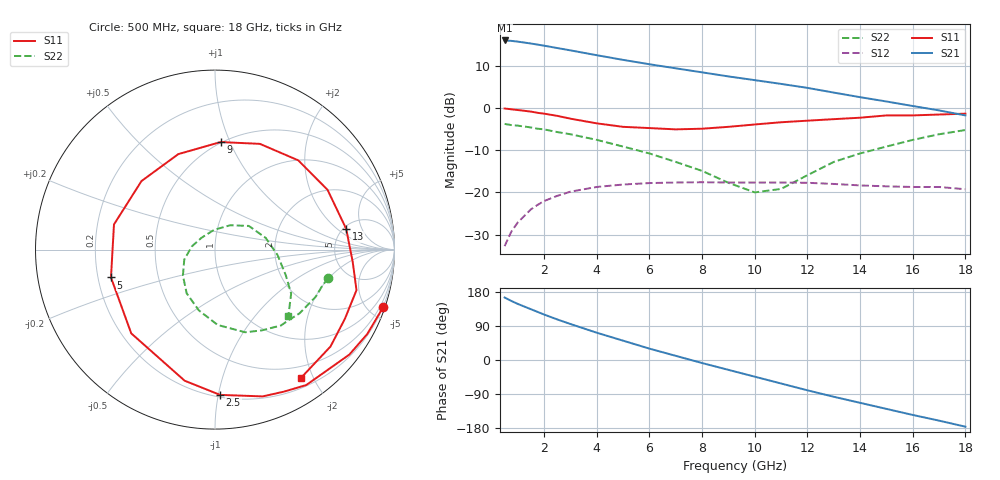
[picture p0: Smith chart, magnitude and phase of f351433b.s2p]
!ATF-35143
!S-PARAMETERS at Vds=3V  Id=10mA.  LAST UPDATED 06-3-99
# ghz s ma r 50
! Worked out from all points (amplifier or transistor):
!   23 points, 500 MHz to 18 GHz, reference 50 ohm
!   highest |S21| = 16.1 dB at 500 MHz (marker M1)
!   |S21| within 3 dB of that: start of sweep to 3.563 GHz
!   unconditionally stable (mu >= 1): 7.966 GHz to end of sweep
!   at 1.5 GHz: K = 0.23, MSG = 19.7 dB, |S12| = -24.0 dB
!   at 7 GHz: K = 0.91, MSG = 13.6 dB, |S12| = -17.7 dB
!   at 18 GHz: K = 1.40, MAG = 5.0 dB, |S12| = -19.3 dB
!   lowest NFmin = 0.12 dB at 500 MHz
!   S11 on the Smith chart (normalised r, x): 500 MHz: 0.18, -5.97; 2.5 GHz: 0.21, -1.01; 5 GHz: 0.25, -0.12; 9 GHz: 0.49, +0.92; 13 GHz: 5.27, +2.70; 18 GHz: 0.33, -1.83
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0.5  0.99 -19.0  6.36 165.0  0.023 77.0  0.65 -14.0
0.75  0.97 -29.0  6.29 156.0  0.034 70.0  0.63 -19.0
1  0.95 -38.0  6.16 148.0  0.044 65.0  0.62 -25.0
1.5  0.91 -56.0  5.85 134.0  0.063 54.0  0.59 -37.0
1.75  0.88 -64.0  5.68 127.0  0.071 49.0  0.57 -43.0
2  0.86 -72.0  5.51 120.0  0.079 44.0  0.56 -49.0
2.5  0.81 -88.0  5.17 107.0  0.091 35.0  0.52 -60.0
3  0.75 -103.0  4.85 95.0  0.102 26.0  0.49 -70.0
4  0.66 -135.0  4.25 72.0  0.116 10.0  0.42 -88.0
5  0.6 -165.0  3.74 51.0  0.124 -5.0  0.35 -105.0
6  0.58 166.0  3.32 30.0  0.129 -19.0  0.29 -123.0
7  0.56 137.0  2.97 11.0  0.131 -32.0  0.23 -141.0
8  0.57 111.0  2.66 -8.0  0.132 -44.0  0.18 -162.0
9  0.6 87.0  2.38 -26.0  0.131 -55.0  0.13 172.0
10  0.64 67.0  2.15 -44.0  0.131 -65.0  0.1 139.0
11  0.68 47.0  1.94 -62.0  0.131 -76.0  0.11 93.0
12  0.71 28.0  1.74 -80.0  0.13 -87.0  0.16 58.0
13  0.74 9.0  1.53 -97.0  0.126 -99.0  0.23 35.0
14  0.77 -5.0  1.35 -113.0  0.121 -107.0  0.29 13.0
15  0.82 -16.0  1.2 -129.0  0.118 -117.0  0.35 -5.0
16  0.82 -28.0  1.06 -145.0  0.116 -126.0  0.42 -20.0
18  0.86 -56.0  0.82 -176.0  0.109 -146.0  0.55 -42.0
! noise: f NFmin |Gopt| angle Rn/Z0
0.5  0.12  0.87  5  0.21
0.9  0.16  0.82  13  0.19
1.5  0.22  0.75  26  0.17
1.8  0.26  0.71  32  0.16
2.5  0.33  0.62  48  0.14
3  0.39  0.57  60  0.13
5  0.6  0.43  114  0.08
6  0.71  0.38  144  0.05
8  0.92  0.34  -151  0.07
10  1.13  0.35  -83  0.21
